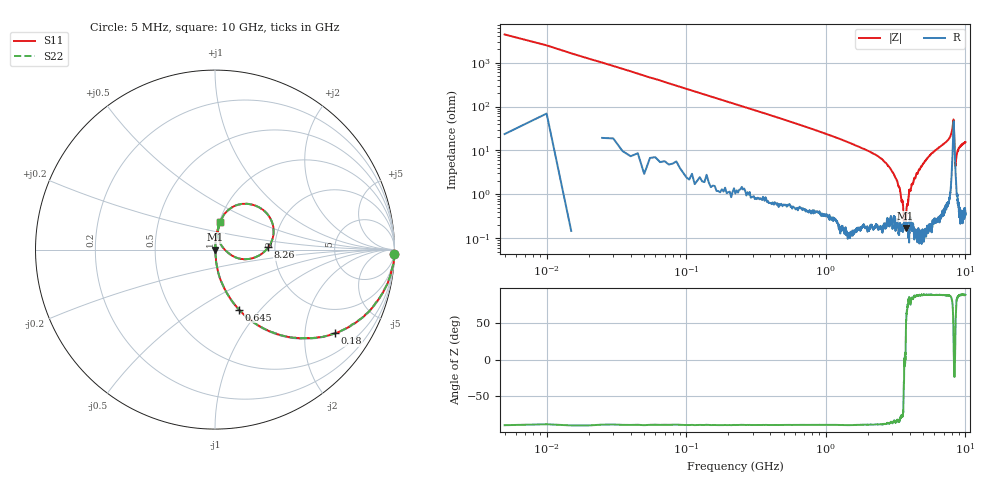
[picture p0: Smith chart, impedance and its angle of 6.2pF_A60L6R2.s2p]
! Amotech Co.,Ltd.
! http://www.amotech.co.kr/
! Part Number: A60L6R2
! These Parameters are Measured in Series Mode Connection
! Operation Temp=25[degC], DC Bias Voltage=0[V]
! Freq. Start=5[MHz] Stop=10[GHz], 2000[Steps]
! Date: Monday, July 14, 2020, 09:33:11
# GHZ S RI R 50.000000
!Freq.(Hz) S11(Real) S11(Imag) S21(Real) S21(Imag) S12(Real) S12(Imag) S22(Real) S22(Imag)
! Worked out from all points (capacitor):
!   2000 points, 5 MHz to 10 GHz, reference 50 ohm
!   read as one part in series: C = 6.26 pF near 55 MHz
!   lowest |Z| = 172 mohm at 3.725 GHz (marker M1)
!   series resonance near 3.649 GHz, so ESL is about 300 pH
!   S11 on the Smith chart (normalised r, x): 5 MHz: 1, -87; 180 MHz: 1.03, -2.85; 645 MHz: 1.01, -0.78; 8.26 GHz: 1.84, +0.05; 10 GHz: 1.01, +0.31
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0.005  0.9994 -0.0229  0.000647 0.0229  0.000647 0.0229  0.9994 -0.0229
0.08  0.9059 -0.2841  0.0941 0.2841  0.0941 0.2841  0.9059 -0.2841
0.18  0.6684 -0.4662  0.3316 0.4662  0.3316 0.4662  0.6684 -0.4662
0.38  0.3126 -0.4586  0.6874 0.4586  0.6874 0.4586  0.3126 -0.4586
0.645  0.1341 -0.3342  0.8659 0.3342  0.8659 0.3342  0.1341 -0.3342
1.675  0.0173 -0.1239  0.9827 0.1239  0.9827 0.1239  0.0173 -0.1239
2.7  0.00434 -0.0513  0.9957 0.0513  0.9957 0.0513  0.00434 -0.0513
3.34  0.00165 -0.0146  0.9983 0.0146  0.9983 0.0146  0.00165 -0.0146
3.55  0.0015 -0.00676  0.9985 0.00676  0.9985 0.00676  0.0015 -0.00676
3.67  0.00219 -0.000117  0.9978 0.000117  0.9978 0.000117  0.00219 -0.000117
3.725  0.00171 0.000216  0.9983 -0.000216  0.9983 -0.000216  0.00171 0.000216
3.81  0.00209 0.005  0.9979 -0.005  0.9979 -0.005  0.00209 0.005
3.985  0.00254 0.0124  0.9975 -0.0124  0.9975 -0.0124  0.00254 0.0124
5.005  0.00362 0.0506  0.9964 -0.0506  0.9964 -0.0506  0.00362 0.0506
6.67  0.0186 0.1233  0.9814 -0.1233  0.9814 -0.1233  0.0186 0.1233
7.675  0.0418 0.1806  0.9582 -0.1806  0.9582 -0.1806  0.0418 0.1806
8.1  0.1635 0.2555  0.8365 -0.2555  0.8365 -0.2555  0.1635 0.2555
8.26  0.2969 0.0125  0.7031 -0.0125  0.7031 -0.0125  0.2969 0.0125
8.335  0.144 -0.0517  0.856 0.0517  0.856 0.0517  0.144 -0.0517
8.485  0.034 0.0252  0.966 -0.0252  0.966 -0.0252  0.034 0.0252
8.94  0.0171 0.1082  0.9829 -0.1082  0.9829 -0.1082  0.0171 0.1082
10  0.0271 0.1516  0.9729 -0.1516  0.9729 -0.1516  0.0271 0.1516
